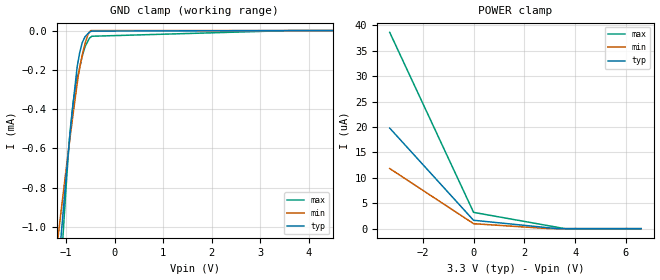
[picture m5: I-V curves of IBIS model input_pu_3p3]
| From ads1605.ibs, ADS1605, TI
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|   INPUT_PU 3.3V Model
[Model]   input_pu_3p3
Model_type   Input
Vinl = 0.99
Vinh = 2.31
|   typ   min   max
|   (nom PVT)   (Fast PVT)   (Slow PVT)
C_comp   4.101e-13   3.469e-13   4.872e-13
|Where nom PVT is NOM Process, 3.3V,39C
|   Fast PVT is Strong Process, 3.6V, -40C
|   Slow PVT is Weak Process, 3.0V, 99C
[Model Spec]
Vinl   0.99   0.9   1.08
Vinh   2.31   2.1   2.52
[Voltage Range]   3.3   3   3.6
|Ambient Temperature   25   85   -40
|Junction Temperature
[Temperature Range]   39   99   -40
[Power Clamp Reference]   3.3   3   3.6
[GND Clamp Reference]   0   0   0
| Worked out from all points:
|   GND clamp passes 1 mA (typ) near -1.09 V on its own axis
[GND Clamp]
|   Voltage   I(typ)   I(min)   I(max)
-3.3V     -8mA       -5.73mA    -13.12mA
-1.168V   -1.231mA   -1.051mA   -1.508mA
-1.116V   -1.076mA   -941.4uA   -1.257mA
-1.068V   -936.5uA   -842.1uA   -1.052mA
-938.4mV  -572.3uA   -578.6uA   -565.9uA
-909.6mV  -498.7uA   -522.7uA   -487.8uA
-852mV    -358.6uA   -413.2uA   -358.6uA
-775.5mV  -186.4uA   -272.9uA   -244.3uA
-669.9mV  -61.53uA   -125.7uA   -130.7uA
-555mV    -16.3uA    -21.98uA   -54.46uA
-498mV    -5.202uA   0A         -33.86uA
6.6V      0A         0A         0A
[POWER Clamp]
|   Voltage   I(typ)   I(min)   I(max)
-3.3V     19.79uA    11.83uA    38.63uA
1.2mV     1.649uA    982.3nA    3.207uA
3V        149.9nA    0A         535.5nA
3.601V    0A         0A         0A
6.6V      0A         0A         0A
